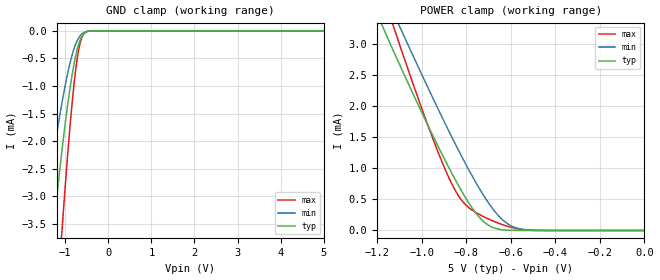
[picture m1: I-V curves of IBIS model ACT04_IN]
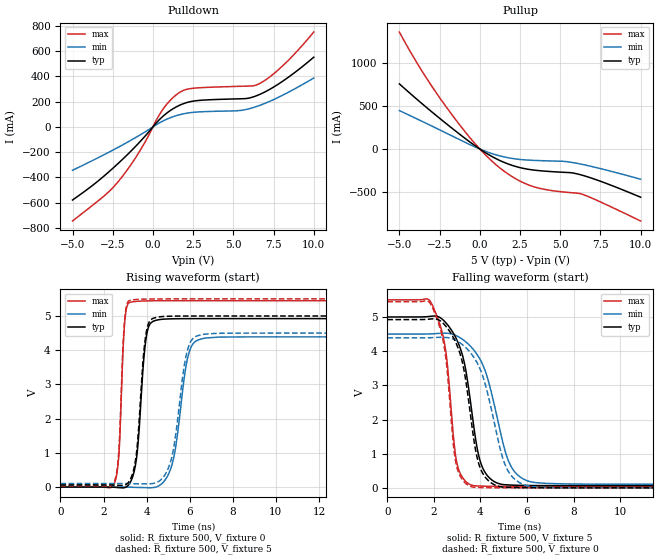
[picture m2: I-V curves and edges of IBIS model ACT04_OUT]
| TEXAS INSTRUMENTS INCORPORATED
| Standard Linear and Logic Group
| IBIS Model of SN74ACT04
| HEX INVERTERS
| This file contains package information for the following:
|  SOIC 14-pin (D) package as [Component] ACT04_D
|  SSOP 14-pin (DB) package as [Component] ACT04_DB
|  PDIP 14-pin (N) package as [Component] ACT04_N
|  TSSOP 14-pin (PW) package as [Component] ACT04_PW
| This device can be powered at the following Vccs:
|  5 volt Vcc
[IBIS Ver]   3.2
[Comment char]  |_char
[File Name]   sn74act04.ibs
[File Rev]   1.1 | a_die
[Date]   August 27, 2002
[Source]   Data created from TI-SPICE simulations at TI-SLL.
[Notes]   The following is an IBIS list for the SN74ACT04.
   Please contact sllibis@ti.com with questions and
   comments concerning SLL IBIS models.
   This IBIS model is created from a BA (back annotated netlist).
[Disclaimer] Property of Texas Instruments Incorporated.  Unauthorized
   reproduction and/or distribution is strictly prohibited.
   This product is protected under copyright law.
   Created 2002, (C) Copyright 2002, Texas Instruments
   Incorporated, All Rights Reserved
   UNLESS THERE IS A SIGNED, WRITTEN AGREEMENT TO THE
   CONTRARY, TEXAS INSTRUMENTS (TI) IS PROVIDING THE IBIS
   MODELS  AND WITHOUT ANY WARRANTY, EXPRESSED OR
   IMPLIED. TI assumes no liability for:
   1) the accuracy of the IBIS models provided to your
   company;
   2) the proper functioning of these IBIS Models in your
   design or for any resulting applications; or
   3) infringement of patents, copyrights or intellectual
   property rights resulting from your use of these IBIS
   models.
   TI provides IBIS Models as a service to our customers.
   You and your company shall not distribute, sell or give
   these models to anyone else without prior written
   permission from TI.
   TI reserves the right to make changes to our products or
   to discontinue any semiconductor product or service
   without notice, and advises our customers to obtain the
   latest version of relevant information to verify, before
   placing orders, that the information being relied on is
   current.
   Please be aware that your receipt and use of the IBIS
   information provided shall serve as acceptance of these
   terms and conditions.  If you do not accept these terms,
   you should return or destroy the IBIS models and any
   other accompanying information immediately.
| Component ACT04_D 14-pin SOIC
[Component]   ACT04_D
[Manufacturer]  Texas Instruments, Inc.
[Package]
|   typ   min   max
R_pkg   3.100e-02   2.800e-02   3.400e-02
L_pkg   3.109e-09   2.462e-09   3.889e-09
C_pkg   4.730e-13   3.630e-13   6.280e-13
[Pin]   signal_name   model_name   R_pin   L_pin   C_pin
1   1A   ACT04_IN   3.300e-02   3.854e-09   6.220e-13
2   1Y   ACT04_OUT   3.200e-02   3.188e-09   4.730e-13
3   2A   ACT04_IN   2.800e-02   2.462e-09   3.770e-13
4   2Y   ACT04_OUT   3.100e-02   2.596e-09   3.630e-13
5   3A   ACT04_IN   2.800e-02   2.521e-09   3.720e-13
6   3Y   ACT04_OUT   3.400e-02   3.250e-09   4.760e-13
7   GND   GND   3.400e-02   3.889e-09   6.280e-13
8   4Y   ACT04_OUT   3.400e-02   3.889e-09   6.280e-13
9   4A   ACT04_IN   3.400e-02   3.250e-09   4.760e-13
10   5Y   ACT04_OUT   2.800e-02   2.521e-09   3.720e-13
11   5A   ACT04_IN   3.100e-02   2.596e-09   3.640e-13
12   6Y   ACT04_OUT   2.800e-02   2.462e-09   3.770e-13
13   6A   ACT04_IN   3.200e-02   3.188e-09   4.730e-13
14   VCC   POWER   3.300e-02   3.854e-09   6.220e-13
| Component ACT04_DB 14-pin SSOP
[Component]   ACT04_DB
[Manufacturer]  Texas Instruments, Inc.
[Package]
|   typ   min   max
R_pkg   4.400e-02   4.100e-02   4.600e-02
L_pkg   3.551e-09   3.258e-09   3.927e-09
C_pkg   4.020e-13   3.600e-13   4.210e-13
[Pin]   signal_name   model_name   R_pin   L_pin   C_pin
1   1A   ACT04_IN   4.600e-02   3.927e-09   4.080e-13
2   1Y   ACT04_OUT   4.400e-02   3.587e-09   4.210e-13
3   2A   ACT04_IN   4.100e-02   3.289e-09   3.980e-13
4   2Y   ACT04_OUT   4.200e-02   3.258e-09   3.600e-13
5   3A   ACT04_IN   4.100e-02   3.286e-09   4.030e-13
6   3Y   ACT04_OUT   4.400e-02   3.586e-09   4.210e-13
7   GND   GND   4.600e-02   3.927e-09   4.080e-13
8   4Y   ACT04_OUT   4.600e-02   3.927e-09   4.080e-13
9   4A   ACT04_IN   4.400e-02   3.586e-09   4.210e-13
10   5Y   ACT04_OUT   4.100e-02   3.286e-09   4.030e-13
11   5A   ACT04_IN   4.300e-02   3.258e-09   3.600e-13
12   6Y   ACT04_OUT   4.100e-02   3.289e-09   3.980e-13
13   6A   ACT04_IN   4.400e-02   3.587e-09   4.210e-13
14   VCC   POWER   4.600e-02   3.927e-09   4.080e-13
| Component ACT04_N 14-pin PDIP
[Component]   ACT04_N
[Manufacturer]   Texas Instruments, Inc.
[Package]
|   typ   min   max
R_pkg   4.500e-02   3.700e-02   6.300e-02
L_pkg   5.407e-09   3.922e-09   6.942e-09
C_pkg   3.890e-13   2.050e-13   6.040e-13
[Pin]   signal_name   model_name   R_pin   L_pin   C_pin
1   1A   ACT04_IN   6.300e-02   6.942e-09   6.040e-13
2   1Y   ACT04_OUT   3.700e-02   6.200e-09   4.060e-13
3   2A   ACT04_IN   4.200e-02   4.389e-09   3.220e-13
4   2Y   ACT04_OUT   3.800e-02   3.922e-09   2.050e-13
5   3A   ACT04_IN   3.900e-02   4.301e-09   2.980e-13
6   3Y   ACT04_OUT   3.800e-02   5.329e-09   3.560e-13
7   GND   GND   5.300e-02   6.510e-09   5.440e-13
8   4Y   ACT04_OUT   5.300e-02   6.437e-09   5.390e-13
9   4A   ACT04_IN   3.900e-02   5.352e-09   3.470e-13
10   5Y   ACT04_OUT   4.200e-02   4.473e-09   2.970e-13
11   5A   ACT04_IN   4.400e-02   4.326e-09   2.250e-13
12   6Y   ACT04_OUT   4.200e-02   4.295e-09   2.800e-13
13   6A   ACT04_IN   4.200e-02   6.318e-09   4.180e-13
14   VCC   POWER   6.100e-02   6.900e-09   6.030e-13
| Component ACT04_PW 14-pin TSSOP
[Component]   ACT04_PW
[Manufacturer]  Texas Instruments, Inc.
[Package]
|   typ   min   max
R_pkg   3.200e-02   2.900e-02   3.500e-02
L_pkg   2.378e-09   2.170e-09   2.680e-09
C_pkg   3.140e-13   2.700e-13   3.350e-13
[Pin]   signal_name   model_name   R_pin   L_pin   C_pin
1   1A   ACT04_IN   3.300e-02   2.618e-09   3.300e-13
2   1Y   ACT04_OUT   3.100e-02   2.313e-09   3.170e-13
3   2A   ACT04_IN   3.000e-02   2.310e-09   3.140e-13
4   2Y   ACT04_OUT   3.100e-02   2.173e-09   2.720e-13
5   3A   ACT04_IN   3.000e-02   2.204e-09   3.090e-13
6   3Y   ACT04_OUT   3.200e-02   2.315e-09   3.170e-13
7   GND   GND   3.500e-02   2.680e-09   3.350e-13
8   4Y   ACT04_OUT   3.300e-02   2.640e-09   3.330e-13
9   4A   ACT04_IN   3.400e-02   2.347e-09   3.190e-13
10   5Y   ACT04_OUT   2.900e-02   2.277e-09   3.130e-13
11   5A   ACT04_IN   3.100e-02   2.170e-09   2.700e-13
12   6Y   ACT04_OUT   3.100e-02   2.244e-09   3.110e-13
13   6A   ACT04_IN   3.300e-02   2.343e-09   3.210e-13
14   VCC   POWER   3.500e-02   2.657e-09   3.320e-13
| Models and submodels in the file (2): ACT04_IN (Input), ACT04_OUT (Output)
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| Model ACT04_IN
| Model ACT04_OUT
[Model]   ACT04_IN
Model_type  Input
Vinl = 0.8
Vinh = 2.0
| variable   typ   min   max
C_comp   4.5pF   NA   NA
[Temperature Range]   40   100   -40
| Ambient temperature   25   85   -40
[Voltage range]   5   4.5   5.5
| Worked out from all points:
|   GND clamp passes 1 mA (typ) near -0.88 V on its own axis
|   POWER clamp passes 1 mA (typ) near -0.88 V on its own axis
[GND Clamp]
| ACT04_IN
|   Voltage   I(typ)   I(min)   I(max)
-5V       -46.92mA   -30.58mA   -59.62mA
-1.56V    -6.035mA   -3.826mA   -9.528mA
-1.51V    -5.59mA    -3.537mA   -8.882mA
-1.305V   -3.869mA   -2.418mA   -6.312mA
-1.255V   -3.478mA   -2.163mA   -5.708mA
-1.08V    -2.21mA    -1.334mA   -3.692mA
-1.06V    -2.076mA   -1.247mA   -3.474mA
-900mV    -1.111mA   -628.4uA   -1.852mA
-770mV    -508.4uA   -270.1uA   -799.3uA
-670mV    -203.9uA   -108.8uA   -280.1uA
-550mV    -38.99uA   -24.34uA   -40.29uA
5V        16.38nA    4.859uA    150.6nA
[POWER Clamp]
| ACT04_IN
|   Voltage   I(typ)   I(min)   I(max)
-5V       45.74mA    45.24mA    49.64mA
-1.17V    3.235mA    3.838mA    3.746mA
-1.125V   2.87mA     3.482mA    3.262mA
-1.075V   2.477mA    3.09mA     2.732mA
-965mV    1.638mA    2.244mA    1.62mA
-895mV    1.129mA    1.722mA    985.3uA
-840mV    755.6uA    1.327mA    587.5uA
-785mV    423.6uA    951.8uA    357.6uA
-695mV    72.53uA    417uA      176.8uA
-640mV    12.79uA    181.6uA    97.2uA
-585mV    1.851uA    53.91uA    37.94uA
-84.45fV  16.38nA    947.5pA    229.7nA
[Model]   ACT04_OUT
Model_type  Output
Vref =   0
Rref =   500
Cref =   50p
Vmeas =   1.5
| variable   typ   min   max
C_comp   10.54pF   6.69pF   16.90pF
| C_pullup   9.47pF   6.98pF   12.15pF
| C_pulldown   11.61pF   6.69pF   16.90pF
[Temperature Range]   40   100   -40
| Ambient temperature   25   85   -40
[Voltage range]   5   4.5   5.5
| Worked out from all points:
|   slope of the pulldown table from 0 to 0.75 V, typ, clamps not added: 7.63 ohm
|   slope of the pullup table from 0 to 0.75 V, typ, clamps not added: 8.61 ohm
|   rising waveform, R_fixture 500, V_fixture 0: 20-80 % time 341ps typ, 559ps min, 208ps max; typ from 0 V to 4.92 V
|   falling waveform, R_fixture 500, V_fixture 5: 20-80 % time 722ps typ, 1.02ns min, 493ps max; typ from 5 V to 0.063 V
|   rising waveform, R_fixture 500, V_fixture 5: 20-80 % time 340ps typ, 561ps min, 208ps max; typ from 0.063 V to 5 V
|   falling waveform, R_fixture 500, V_fixture 0: 20-80 % time 708ps typ, 992ps min, 486ps max; typ from 4.92 V to 0 V
[Pulldown]
| ACT04_OUT
|   Voltage   I(typ)   I(min)   I(max)
-5V       -580.4mA   -344.3mA   -746.8mA
-3V       -385.5mA   -218.2mA   -544mA
-2.13V    -286.2mA   -159.9mA   -429.7mA
-860mV    -125.1mA   -68.18mA   -200.6mA
550mV     75.78mA    41.96mA    126.1mA
1.45V     158.6mA    88.99mA    254.7mA
1.895V    184.2mA    103.6mA    289.5mA
2.39V     202mA      113.9mA    304.9mA
5.385V    222.9mA    129.9mA    322.1mA
6.535V    252.1mA    165.9mA    338.3mA
8.04V     360.1mA    249.9mA    481.5mA
10V       553.1mA    387.7mA    752.8mA
[Pullup]
| ACT04_OUT
|   Voltage   I(typ)   I(min)   I(max)
-5V       757.2mA    446.5mA    1.36A
-3.49V    510.8mA    312.3mA    875.4mA
-1.795V   251.3mA    158mA      414.2mA
-115mV    14.91mA    9.349mA    23.63mA
600mV     -71.21mA   -43.73mA   -114.4mA
1.315V    -140mA     -83.59mA   -230.4mA
2.33V     -208.6mA   -118.5mA   -356.8mA
3.345V    -245mA     -132.5mA   -438.6mA
5.24V     -271.7mA   -144.4mA   -501mA
6.195V    -296.4mA   -172.6mA   -517.7mA
7.675V    -387.4mA   -236.4mA   -631mA
10V       -561.1mA   -352.2mA   -838mA
[Ramp]
| ACT04_OUT
| variable   typ   min   max
dV/dt_r   2.97/3.51E-10   2.65/5.67E-10   3.28/2.14E-10
dV/dt_f   2.98/7.37E-10   2.65/1.03E-09   3.29/5.02E-10
R_load = 500
[Rising Waveform]
| ACT04_OUT
R_fixture =   500
C_fixture =   0
L_fixture =   0
V_fixture =   0
V_fixture_min = 0
V_fixture_max = 0
|   Time   V(typ)   V(min)   V(max)
0s        1.299nV    2.226nV    795.2pV
2.51ns    -5.544mV   365.7uV    116.8mV
2.72ns    -15.92mV   260.9uV    1.012V
3ns       -11.66mV   -1.136mV   4.928V
3.335ns   268.9mV    -5.766mV   5.414V
3.99ns    4.407V     -16.99mV   5.44V
4.575ns   4.893V     38.66mV    5.445V
5.985ns   4.922V     3.963V     5.446V
6.745ns   4.923V     4.356V     5.446V
50ns      4.923V     4.389V     5.446V
[Falling Waveform]
| ACT04_OUT
R_fixture =   500
C_fixture =   0
L_fixture =   0
V_fixture =   5
V_fixture_min = 4.5
V_fixture_max = 5.5
|   Time   V(typ)   V(min)   V(max)
0s        5V         4.5V       5.5V
1.95ns    5.027V     4.507V     5.326V
2.5ns     4.841V     4.524V     4.053V
2.995ns   4.318V     4.442V     707.8mV
3.335ns   3.572V     4.292V     211.2mV
3.705ns   1.842V     4.041V     65.67mV
4.385ns   291.8mV    3.017V     45.72mV
5.26ns    83.64mV    702.9mV    41.57mV
6.35ns    67.18mV    154mV      40.86mV
50ns      63.36mV    104.1mV    40.77mV
[Rising Waveform]
| ACT04_OUT
R_fixture =   500
C_fixture =   0
L_fixture =   0
V_fixture =   5
V_fixture_min = 4.5
V_fixture_max = 5.5
|   Time   V(typ)   V(min)   V(max)
0s        63.36mV    104.1mV    40.77mV
2.51ns    58.06mV    104.4mV    166.2mV
2.715ns   49.67mV    104.2mV    1.075V
2.985ns   56.5mV     103mV      4.921V
3.26ns    245.5mV    99.95mV    5.463V
3.98ns    4.512V     95.45mV    5.494V
4.55ns    4.97V      160.2mV    5.498V
5.92ns    4.999V     4.052V     5.5V
6.665ns   5V         4.467V     5.5V
50ns      5V         4.5V       5.5V
[Falling Waveform]
| ACT04_OUT
R_fixture =   500
C_fixture =   0
L_fixture =   0
V_fixture =   0
V_fixture_min = 0
V_fixture_max = 0
|   Time   V(typ)   V(min)   V(max)
0s        4.923V     4.389V     5.446V
1.94ns    4.945V     4.396V     5.273V
2.47ns    4.764V     4.402V     4.021V
2.97ns    4.209V     4.309V     652.3mV
3.295ns   3.439V     4.151V     179.5mV
3.69ns    1.539V     3.845V     21.45mV
4.145ns   372.7mV    3.176V     6.949mV
5.1ns     16.5mV     610.4mV    917.5uV
6.22ns    2.722mV    33.8mV     108.9uV
50ns      -3.195nV   -3.043nV   -16.38nV
